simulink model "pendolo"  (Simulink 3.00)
settings: Solver=ode45  StartTime=0  StopTime=10000  FixedStep=0.1  MaxStep=0.1  RelTol=1e-3  AbsTol=1e-3
undefined symbols (not defined in the file or in its folder): h, l, m

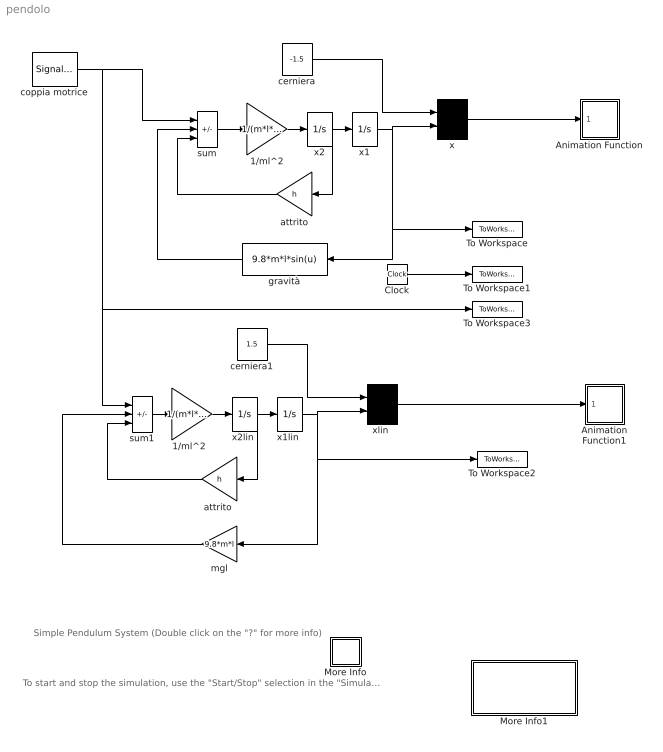
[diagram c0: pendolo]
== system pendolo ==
  note: To start and stop the simulation, use the "Start/Stop" selection in the "Simulation" pull-down menu
  note: Simple Pendulum System (Double click on the "?" for more info)
  1/ml^2 : Gain  Gain=1/(m*l*l)  SaturateOnIntegerOverflow=on
  "1/ml^2  " : Gain  Gain=1/(m*l*l)  SaturateOnIntegerOverflow=on
  Animation Function : Subsystem  mask(Animation Block){ts=0.02}
      mask prompts: ts "Sample time:"
  Animation Function1 : Subsystem  mask(Animation Block){ts=0.02}
      mask prompts: ts "Sample time:"
  Clock : Clock
  More Info : Subsystem
  More Info1 : Subsystem
  To Workspace : ToWorkspace  VariableName=y  SampleTime=0  SaveFormat=Matrix
  To Workspace1 : ToWorkspace  VariableName=t  SampleTime=0  SaveFormat=Matrix
  To Workspace2 : ToWorkspace  VariableName=ylin  SampleTime=0  SaveFormat=Matrix
  To Workspace3 : ToWorkspace  VariableName=c  SampleTime=0  SaveFormat=Matrix
  attrito : Gain  Orientation=left  Gain=h  SaturateOnIntegerOverflow=on
  "attrito " : Gain  Orientation=left  Gain=h  SaturateOnIntegerOverflow=on
  cerniera : Constant  Value=-1.5
  cerniera1 : Constant  Value=1.5
  coppia motrice : SignalGenerator  WaveForm=square  Amplitude=4.000000  Frequency=1.000000  Units=rad/sec
  gravità : Fcn  Orientation=left  Expr=9.8*m*l*sin(u)
  mgl : Gain  Orientation=left  Gain=9.8*m*l  SaturateOnIntegerOverflow=on
  sum : Sum  Inputs=+--  SaturateOnIntegerOverflow=on
  sum1 : Sum  Inputs=+--  SaturateOnIntegerOverflow=on
  x : Mux  Inputs=2
  x1 : Integrator  ExternalReset=none  InitialConditionSource=internal  InitialCondition=0  LimitOutput=off  UpperSaturationLimit=inf  LowerSaturationLimit=-inf  ShowSaturationPort=off  ShowStatePort=off  AbsoluteTolerance=auto
  "x1lin " : Integrator  ExternalReset=none  InitialConditionSource=internal  InitialCondition=0  LimitOutput=off  UpperSaturationLimit=inf  LowerSaturationLimit=-inf  ShowSaturationPort=off  ShowStatePort=off  AbsoluteTolerance=auto
  x2 : Integrator  ExternalReset=none  InitialConditionSource=internal  InitialCondition=0  LimitOutput=off  UpperSaturationLimit=inf  LowerSaturationLimit=-inf  ShowSaturationPort=off  ShowStatePort=off  AbsoluteTolerance=auto
  "x2lin " : Integrator  ExternalReset=none  InitialConditionSource=internal  InitialCondition=0  LimitOutput=off  UpperSaturationLimit=inf  LowerSaturationLimit=-inf  ShowSaturationPort=off  ShowStatePort=off  AbsoluteTolerance=auto
  "xlin " : Mux  Inputs=2
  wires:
  x2/1 -> attrito/1, x1/1
  cerniera/1 -> x/1
  x1/1 -> x/2, gravità/1, To Workspace/1
  gravità/1 -> sum/2
  Clock/1 -> To Workspace1/1
  "attrito "/1 -> sum1/3
  "x2lin "/1 -> "attrito "/1, "x1lin "/1
  cerniera1/1 -> "xlin "/1
  "x1lin "/1 -> "xlin "/2, To Workspace2/1, mgl/1
  mgl/1 -> sum1/2
  1/ml^2/1 -> x2/1
  sum/1 -> 1/ml^2/1
  attrito/1 -> sum/3
  coppia motrice/1 -> sum1/1, To Workspace3/1, sum/1
  "1/ml^2  "/1 -> "x2lin "/1
  sum1/1 -> "1/ml^2  "/1
  "xlin "/1 -> Animation Function1/1(In1)
  x/1 -> Animation Function/1(In1)

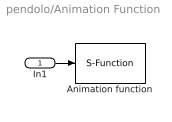
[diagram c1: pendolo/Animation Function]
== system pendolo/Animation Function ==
  In1 : Inport  Port=1  PortWidth=-1  SampleTime=-1  DataType=auto
  Animation function : S-Function  FunctionName=pndanim1  Parameters=ts  PortCounts=[]  SFunctionModules=''
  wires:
  In1/1 -> Animation function/1

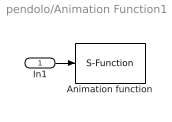
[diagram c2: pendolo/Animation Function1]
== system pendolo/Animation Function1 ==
  In1 : Inport  Port=1  PortWidth=-1  SampleTime=-1  DataType=auto
  Animation function : S-Function  FunctionName=pndanim1  Parameters=ts  PortCounts=[]  SFunctionModules=''
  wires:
  In1/1 -> Animation function/1

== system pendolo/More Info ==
  note: Associated with the demo is an animation function that will automatically open a figure window and display to it.
  note: This system models a simple pendulum system with an applied external moment that varies periodically.
  note: Try experimenting with different initial conditions and different setting for the applied moment M.

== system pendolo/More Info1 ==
  note: This system models a double pendulum system where the rest state has both pendulums hanging vertically.
  note: Associated with the demo is an animation function that will automatically open a figure window and display to it.
  note: Try experimenting with different initial conditions for alpha and gamma to see the unusal coupling effects.
